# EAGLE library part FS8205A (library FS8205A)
Dual N-Channel Enahncement Mode Power MOSFET Source: Datasheet
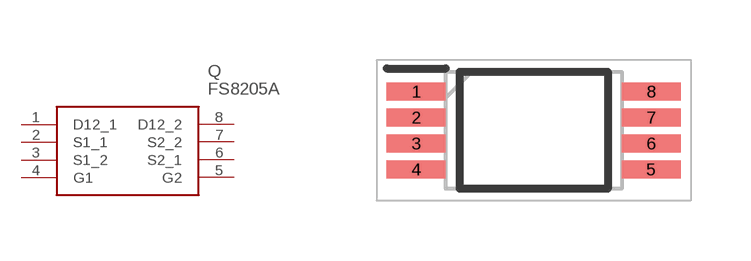
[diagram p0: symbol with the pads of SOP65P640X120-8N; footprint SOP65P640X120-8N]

Designator prefix Q

## FS8205A (Description: Dual N-Channel Enahncement Mode Power MOSFET; Height: 1.2mm; Manufacturer_Name: Fortune Semiconductor Corporation; Manufacturer_Part_Number: FS8205A)  [SOP65P640X120-8N]
1  D12_1
2  S1_1
3  S1_2
4  G1
5  G2
6  S2_1
7  S2_2
8  D12_2

## Footprint SOP65P640X120-8N (pad centres in mm)
FS8205A
smd 1.475 x 0.45: 1 -2.938,0.975; 2 -2.938,0.325; 3 -2.938,-0.325; 4 -2.938,-0.975; 5 2.938,-0.975; 6 2.938,-0.325; 7 2.938,0.325; 8 2.938,0.975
